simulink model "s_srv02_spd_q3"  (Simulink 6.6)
settings: Solver=ode4  SolverMode=SingleTasking  StartTime=0.0  StopTime=5  FixedStep=0.0002  RelTol=1e-3  AbsTol=1e-6
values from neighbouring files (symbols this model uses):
  a = 10^(-21/20)    (= 0.0891250938134)    [d_lag_q3.m]    (also in d_lead.m = (1+sin(phi_m)) / (1-sin(phi_m)); setup_srv02_exp03_spd.m = 1)
  bsp = 0    [setup_srv02_exp03_spd.m]
  IMAX_AMP = 0    [config_srv02.m]
  K = Am / Beq_v    [d_model_param.m]    (also in setup_srv02_exp01_mdl.m = 1)
  Kc = 10^(e_ss_meas/e_ss_min/20)    (= 2.14783047413)    [d_lag_q3.m]    (also in d_lead.m = 53.0884444231; setup_srv02_exp03_spd.m = 0)
  ki = wn^2*tau/K    [d_pi_design.m]    (also in setup_srv02_exp03_spd.m = 0; d_i_design.m = -( -AmpMax + kp * e_ss ) / ti / e_ss; setup_srv02_exp02_pos.m = 0)
  kp = (-1+2*zeta*wn*tau)/K    [d_pi_design.m]    (also in setup_srv02_exp03_spd.m = 0; d_pv_design.m = wn^2/K*tau; setup_srv02_exp02_pos.m = 0)
  T = 10 / (wg_des * a)    [d_lag_q3.m]    (also in d_lead.m = 1 / (w_m * sqrt(a)); setup_srv02_exp03_spd.m = 1)
  VMAX_DAC = 10    [setup_srv02_exp03_spd.m]    (also in setup_srv02_exp01_mdl.m; setup_srv02_exp02_pos.m)
undefined symbols (not defined in the file or in its folder): square
libraries: simulink x3

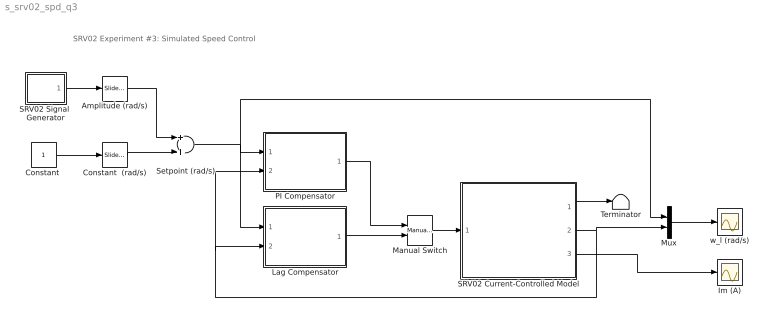
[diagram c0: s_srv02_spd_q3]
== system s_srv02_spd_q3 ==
  note: SRV02 Experiment #3: Simulated Speed Control
  Amplitude (rad/s) : simulink/Math Operations/Slider Gain  SystemSampleTime=-1  low=0  gain=2.5  high=10
  "Constant " : Constant
  Constant  (rad/s) : simulink/Math Operations/Slider Gain  SystemSampleTime=-1  low=0  gain=5  high=10
  Im (A) : Scope
  Lag Compensator : Subsystem
  Manual Switch : simulink/Signal Routing/Manual Switch  SystemSampleTime=-1  sw=1  action=0  varsize=off
  Mux : Mux  Inputs=2
  PI Compensator : Subsystem
  SRV02 Current-Controlled Model : Subsystem
  SRV02 Signal  Generator : Subsystem  mask(QET Signal Generator){sig_type=square, a=1, f=0.4}
      mask prompts: sig_type "Signal Type"; a "Amplitude"; f "Frequency (Hz)"
      mask help: Generates a square, triangular, or sinusoidal waveform of a specified amplitude and frequency.
  Setpoint (rad/s) : Sum  OutScaling=2^-10
  Terminator : Terminator
  w_l (rad/s) : Scope
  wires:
  Setpoint (rad/s)/1 -> Mux/1, PI Compensator/1(wd (rad/s)), Lag Compensator/1(wd (rad/s))
  Manual Switch/1 -> SRV02 Current-Controlled Model/1(I_ref (A))
  SRV02 Current-Controlled Model/2(omega_l (rad/s)) -> Mux/2, PI Compensator/2(wl (rad)), Lag Compensator/2(wl (rad/s))
  Mux/1 -> w_l (rad/s)/1
  SRV02 Current-Controlled Model/3(Im (A)) -> Im (A)/1
  SRV02 Current-Controlled Model/1(theta_l (rad)) -> Terminator/1
  Lag Compensator/1(u) -> Manual Switch/2
  PI Compensator/1(u) -> Manual Switch/1
  SRV02 Signal  Generator/1(out) -> Amplitude (rad/s)/1
  Amplitude (rad/s)/1 -> Setpoint (rad/s)/1
  "Constant "/1 -> Constant  (rad/s)/1
  Constant  (rad/s)/1 -> Setpoint (rad/s)/2

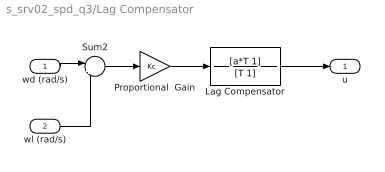
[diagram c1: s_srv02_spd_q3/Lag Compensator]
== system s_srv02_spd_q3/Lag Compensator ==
  wd (rad/s) : Inport
  wl (rad/s) : Inport  Port=2
  Lag Compensator : TransferFcn  Numerator=[a*T 1]  Denominator=[T 1]
  Proportional  Gain : Gain  Gain=Kc
  Sum2 : Sum  Inputs=|+-
  u : Outport
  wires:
  Sum2/1 -> Proportional  Gain/1
  wd (rad/s)/1 -> Sum2/1
  wl (rad/s)/1 -> Sum2/2
  Proportional  Gain/1 -> Lag Compensator/1
  Lag Compensator/1 -> u/1

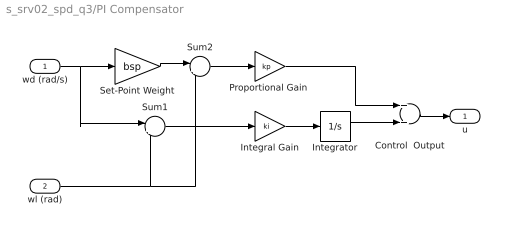
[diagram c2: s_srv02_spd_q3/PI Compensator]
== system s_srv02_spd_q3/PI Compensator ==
  wd (rad/s) : Inport
  wl (rad) : Inport  Port=2
  Control  Output : Sum  OutScaling=2^-10
  Integral Gain : Gain  Gain=ki
  Integrator : Integrator  UpperSaturationLimit=10  LowerSaturationLimit=-10
  "Proportional Gain " : Gain  Gain=kp
  Set-Point Weight : Gain  Gain=bsp
  Sum1 : Sum  Inputs=|+-
  Sum2 : Sum  Inputs=|+-
  u : Outport
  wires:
  Sum1/1 -> Integral Gain/1
  Integral Gain/1 -> Integrator/1
  Integrator/1 -> Control  Output/2
  "Proportional Gain "/1 -> Control  Output/1
  Set-Point Weight/1 -> Sum2/1
  Sum2/1 -> "Proportional Gain "/1
  wd (rad/s)/1 -> Set-Point Weight/1, Sum1/1
  Control  Output/1 -> u/1
  wl (rad)/1 -> Sum1/2, Sum2/2

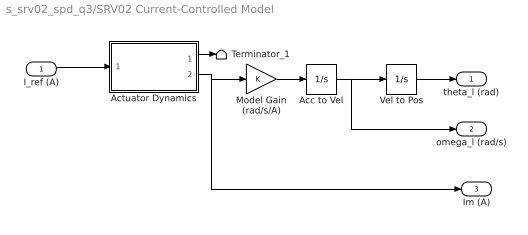
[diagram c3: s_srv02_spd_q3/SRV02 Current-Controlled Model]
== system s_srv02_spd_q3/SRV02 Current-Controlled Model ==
  I_ref (A) : Inport
  Acc to Vel : Integrator
  Actuator Dynamics : Subsystem
  Model Gain (rad/s/A) : Gain  Gain=K
  Terminator_1 : Terminator
  Vel to Pos : Integrator
  theta_l (rad) : Outport
  omega_l (rad/s) : Outport  Port=2
  Im (A) : Outport  Port=3
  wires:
  Acc to Vel/1 -> omega_l (rad/s)/1, Vel to Pos/1
  Model Gain (rad/s/A)/1 -> Acc to Vel/1
  Actuator Dynamics/1(Vdaq (V)) -> Terminator_1/1
  I_ref (A)/1 -> Actuator Dynamics/1(I_ref (A))
  Actuator Dynamics/2(Im (A)) -> Model Gain (rad/s/A)/1, Im (A)/1
  Vel to Pos/1 -> theta_l (rad)/1

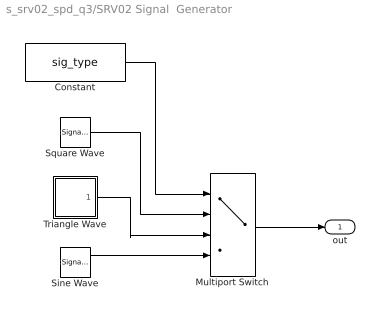
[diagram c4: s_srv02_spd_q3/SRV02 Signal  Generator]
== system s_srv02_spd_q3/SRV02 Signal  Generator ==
  Constant : Constant  Value=sig_type
  Multiport Switch : MultiPortSwitch  Inputs=3
  Sine Wave : SignalGenerator  Amplitude=a  Frequency=f
  Square Wave : SignalGenerator  WaveForm=square  Amplitude=a  Frequency=f
  Triangle Wave : Subsystem
  out : Outport
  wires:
  Square Wave/1 -> Multiport Switch/2
  Triangle Wave/1(out) -> Multiport Switch/3
  Sine Wave/1 -> Multiport Switch/4
  Multiport Switch/1 -> out/1
  Constant/1 -> Multiport Switch/1

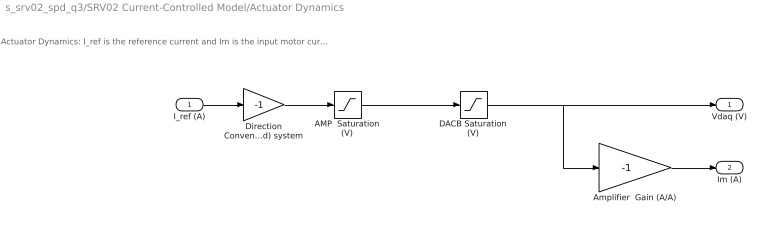
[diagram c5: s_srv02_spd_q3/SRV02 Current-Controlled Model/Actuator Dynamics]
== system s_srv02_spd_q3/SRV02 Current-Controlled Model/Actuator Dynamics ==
  note: Actuator Dynamics: I_ref is the reference current and Im is the input motor current after going through the DACB and amplifier limitiations.
  I_ref (A) : Inport
  AMP  Saturation (V) : Saturate  UpperLimit=IMAX_AMP  LowerLimit=-IMAX_AMP
  Amplifier  Gain (A/A) : Gain  Gain=-1
  DACB Saturation (V) : Saturate  UpperLimit=VMAX_DAC  LowerLimit=-VMAX_DAC
  Direction Convention: (Right-Hand) system : Gain  Gain=-1
  Vdaq (V) : Outport
  Im (A) : Outport  Port=2
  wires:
  I_ref (A)/1 -> Direction Convention: (Right-Hand) system/1
  AMP  Saturation (V)/1 -> DACB Saturation (V)/1
  DACB Saturation (V)/1 -> Amplifier  Gain (A/A)/1, Vdaq (V)/1
  Amplifier  Gain (A/A)/1 -> Im (A)/1
  Direction Convention: (Right-Hand) system/1 -> AMP  Saturation (V)/1

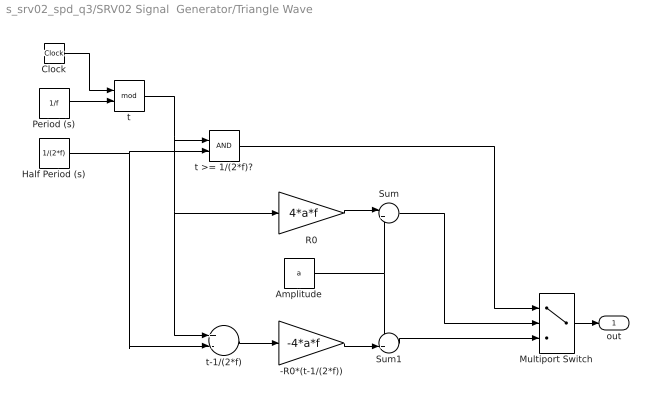
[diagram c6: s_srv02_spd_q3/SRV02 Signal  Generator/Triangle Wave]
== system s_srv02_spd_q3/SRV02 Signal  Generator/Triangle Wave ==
  -R0*(t-1/(2*f)) : Gain  Gain=-4*a*f
  Amplitude : Constant  Value=a
  Clock : Clock
  Half Period (s) : Constant  Value=1/(2*f)
  Multiport Switch : MultiPortSwitch  Inputs=2  zeroidx=on
  Period (s) : Constant  Value=1/f
  R0 : Gain  Gain=4*a*f
  Sum : Sum  Inputs=|+-
  Sum1 : Sum  Inputs=++|
  t : Math  Operator=mod
  t >= 1/(2*f)? : RelationalOperator  LogicOutDataTypeMode=Boolean
  t-1/(2*f) : Sum  Inputs=+-  OutScaling=2^-10
  out : Outport
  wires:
  Sum1/1 -> Multiport Switch/3
  Sum/1 -> Multiport Switch/2
  t >= 1/(2*f)?/1 -> Multiport Switch/1
  -R0*(t-1/(2*f))/1 -> Sum1/2
  Amplitude/1 -> Sum1/1, Sum/2
  R0/1 -> Sum/1
  t-1/(2*f)/1 -> -R0*(t-1/(2*f))/1
  Half Period (s)/1 -> t-1/(2*f)/2, t >= 1/(2*f)?/2
  t/1 -> t-1/(2*f)/1, R0/1, t >= 1/(2*f)?/1
  Period (s)/1 -> t/2
  Clock/1 -> t/1
  Multiport Switch/1 -> out/1
